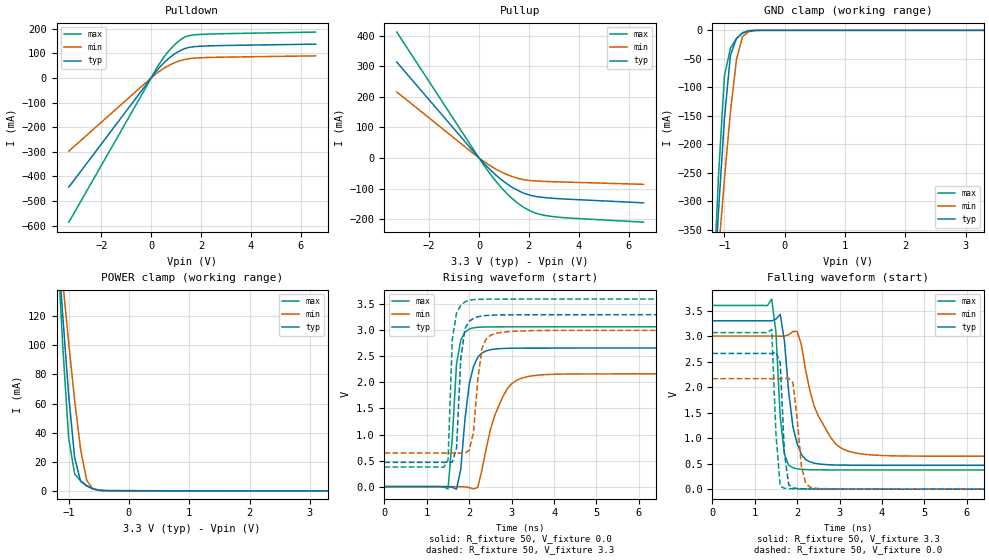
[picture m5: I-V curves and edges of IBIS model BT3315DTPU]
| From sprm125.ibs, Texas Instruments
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[Model]   BT3315DTPU
| I/O WITH PULLUP
Model_type   I/O
Vinh = 2.00
Vinl = 0.80
Enable   Active-Low
Polarity   Non-Inverting
| signals   A, GZ, Y
Vmeas = 1.5
|   typ   min   max
C_comp   1.6130p   1.5354p   1.7989p
|   typ   min   max
[Temperature Range]   25   -40   125
|   typ   min   max
[Voltage Range]   3.30V   3.00V   3.60V
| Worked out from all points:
|   slope of the pulldown table from 0 to 0.495 V, typ, clamps not added: 8.31 ohm
|   slope of the pullup table from 0 to 0.495 V, typ, clamps not added: 11.7 ohm
|   GND clamp passes 1 mA (typ) near -0.60 V on its own axis
|   POWER clamp passes 1 mA (typ) near -0.56 V on its own axis
|   rising waveform, R_fixture 50, V_fixture 0.0: 20-80 % time 227ps typ, 469ps min, 154ps max; typ from 0 V to 2.66 V
|   falling waveform, R_fixture 50, V_fixture 3.3: 20-80 % time 241ps typ, 559ps min, 147ps max; typ from 3.3 V to 0.467 V
|   rising waveform, R_fixture 50, V_fixture 3.3: 20-80 % time 132ps typ, 172ps min, 104ps max; typ from 0.467 V to 3.3 V
|   falling waveform, R_fixture 50, V_fixture 0.0: 20-80 % time 108ps typ, 154ps min, 112ps max; typ from 2.66 V to 0 V
[Pulldown]
|   Voltage   I(typ)   I(min)   I(max)
-3.3V     -443.2mA   -297.4mA   -586.1mA
200mV     26.36mA    16.88mA    36.1mA
600mV     69.79mA    44.5mA     96.01mA
800mV     86.98mA    55.31mA    120.1mA
1.1V      107.3mA    67.84mA    149mA
1.4V      120.9mA    76.06mA    168.2mA
1.9V      128.4mA    81.63mA    176.5mA
6.6V      137.5mA    89.76mA    186.4mA
[GND_clamp]
|   Voltage   I(typ)   I(min)   I(max)
-3.3V     -4.811A    -3.63A     -6.247A
-1.2V     -504.1mA   -527.5mA   -496.6mA
-1.1V     -320mA     -391.3mA   -259mA
-1V       -154.5mA   -261.1mA   -80.07mA
-900mV    -43.32mA   -142.6mA   -30.81mA
-800mV    -14.05mA   -51.16mA   -14.64mA
-700mV    -5.037mA   -10.97mA   -4.191mA
-600mV    -961.5uA   -2.449mA   -466.6uA
-400mV    -4.855uA   -52.49uA   -479.3nA
3.3V      266.4pA    4.204uA    88.82pA
[Pullup]
|   Voltage   I(typ)   I(min)   I(max)
-3.3V     313.3mA    215.7mA    411.3mA
-200mV    18.73mA    12.64mA    24.99mA
300mV     -26.46mA   -17.43mA   -35.88mA
900mV     -71.16mA   -45.96mA   -97.51mA
1.2V      -89.06mA   -56.81mA   -122.9mA
1.5V      -103.8mA   -65.22mA   -144.3mA
1.8V      -115.1mA   -71.07mA   -161.7mA
2.1V      -122.9mA   -74.31mA   -174.7mA
2.7V      -130.1mA   -76.88mA   -188.6mA
3.6V      -134.9mA   -79.19mA   -196.2mA
6.6V      -146.8mA   -86.27mA   -210mA
[POWER_clamp]
|   Voltage   I(typ)   I(min)   I(max)
-3.3V     1.584A     1.199A     2.052A
-1.2V     182.8mA    190mA      180.5mA
-1.1V     122.3mA    145.4mA    101.8mA
-1V       66.45mA    102.4mA    36.68mA
-900mV    22.85mA    62.33mA    11.47mA
-800mV    6.433mA    28.18mA    6.816mA
-700mV    3.2mA      7.14mA     3.571mA
-600mV    1.373mA    1.452mA    1.297mA
-500mV    357.3uA    341.4uA    240.6uA
-400mV    65.6uA     67.61uA    56.84uA
3.3V      -108.3uA   -68.37uA   -162.1uA
[Ramp]
|   I(typ)   I(min)   I(max)
dV/dt_r   1.596/0.221n   1.299/0.470n   1.841/0.134n
dV/dt_f   1.700/0.236n   1.413/0.561n   1.934/0.133n
[Rising Waveform]
R_fixture = 50
V_fixture = 0.0
|  pu_on
|  TIME   V(typ)   V(min)   V(max)
0s        1nV        11nV       1nV
1.5ns     1.189mV    119.9uV    -44.7mV
1.7ns     -48.71mV   522.6uV    2.357V
1.8ns     334.4mV    921.7uV    2.808V
2ns       1.971V     -18.91mV   3.026V
2.2ns     2.484V     -16.74mV   3.058V
2.3ns     2.565V     322.3mV    3.062V
2.6ns     2.64V      1.363V     3.066V
3.2ns     2.658V     2.071V     3.067V
10ns      2.66V      2.165V     3.068V
[Falling Waveform]
R_fixture = 50
V_fixture = 3.3
V_fixture_min = 3.0
V_fixture_max = 3.6
|  pd_on
|  TIME   V(typ)   V(min)   V(max)
0s        3.3V       3V         3.6V
1.4ns     3.298V     3V         3.726V
1.5ns     3.333V     3V         3.07V
1.6ns     3.427V     2.998V     1.421V
1.7ns     2.902V     3V         681.4mV
1.9ns     1.221V     3.09V      419.3mV
2.1ns     678.7mV    2.826V     389.8mV
2.5ns     496.2mV    1.431V     379mV
3.2ns     469.6mV    745.6mV    376.7mV
10ns      466.6mV    645mV      376.2mV
[Rising Waveform]
R_fixture = 50
V_fixture = 3.3
V_fixture_min = 3.0
V_fixture_max = 3.6
|  pd_off
|  TIME   V(typ)   V(min)   V(max)
0s        466.6mV    644.9mV    376.2mV
1.5ns     466mV      645.3mV    511.7mV
1.6ns     469.6mV    645.1mV    2.822V
1.7ns     739.3mV    644.1mV    3.333V
1.8ns     2.445V     641.9mV    3.479V
1.9ns     3.035V     644.6mV    3.547V
2.1ns     3.228V     1.039V     3.59V
2.3ns     3.275V     2.653V     3.596V
2.6ns     3.293V     2.94V      3.598V
10ns      3.3V       3V         3.6V
[Falling Waveform]
R_fixture = 50
V_fixture = 0.0
|  pu_off
|  TIME   V(typ)   V(min)   V(max)
0s        2.66V      2.165V     3.068V
1.4ns     2.658V     2.165V     3.132V
1.5ns     2.683V     2.164V     1.074V
1.6ns     2.487V     2.164V     58.19mV
1.7ns     706mV      2.167V     18.2mV
1.8ns     87.02mV    2.174V     10.21mV
1.9ns     23.64mV    2.084V     6.707mV
2.1ns     9.634mV    444.3mV    3.045mV
2.3ns     5.379mV    41.61mV    1.709mV
10ns      285nV      4.579uV    145nV
